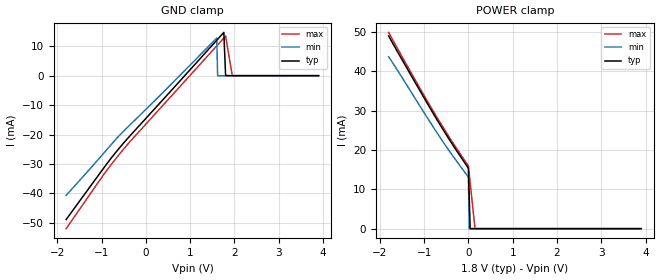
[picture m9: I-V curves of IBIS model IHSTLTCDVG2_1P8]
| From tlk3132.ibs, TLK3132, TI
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|   Model IHSTLTCDVG2_1P8
[Model]   IHSTLTCDVG2_1P8
Model_type   Input
Polarity   Non-Inverting
Vinl =   0.7000V
Vinh =   1.1000V
C_comp   0.7726pF   0.7726pF   0.7726pF
[Temperature Range]   25.0000   0.1250k   -40.0000
[Pullup Reference]   1.8000V   1.6200V   1.9500V
[Pulldown Reference]   0.000V   0.000V   0.000V
[POWER Clamp Reference]   1.8000V   1.6200V   1.9500V
[GND Clamp Reference]   0.000V   0.000V   0.000V
[GND_clamp]
| voltage   I(typ)   I(min)   I(max)
-1.8V     -48.85mA   -40.63mA   -51.96mA
-920mV    -30.72mA   -25.77mA   -32.93mA
-520mV    -23.18mA   -19.09mA   -25.24mA
400mV     -7.911mA   -5.484mA   -9.818mA
1.6V      12.03mA    12.78mA    10.12mA
1.62V     12.36mA    0A         10.45mA
1.76V     14.7mA     0A         12.78mA
1.8V      0A         0A         13.45mA
1.95V     0A         0A         0A
3.9V      0A         0A         0A
[POWER_clamp]
| voltage   I(typ)   I(min)   I(max)
-1.8V     48.95mA    43.68mA    49.85mA
-820mV    29.76mA    26.29mA    30.35mA
-420mV    22.46mA    19.57mA    23.03mA
0V        15.36mA    13.09mA    15.95mA
20mV      7.681mA    0A         13.82mA
40mV      0A         0A         11.7mA
150mV     0A         0A         0A
3.9V      0A         0A         0A
